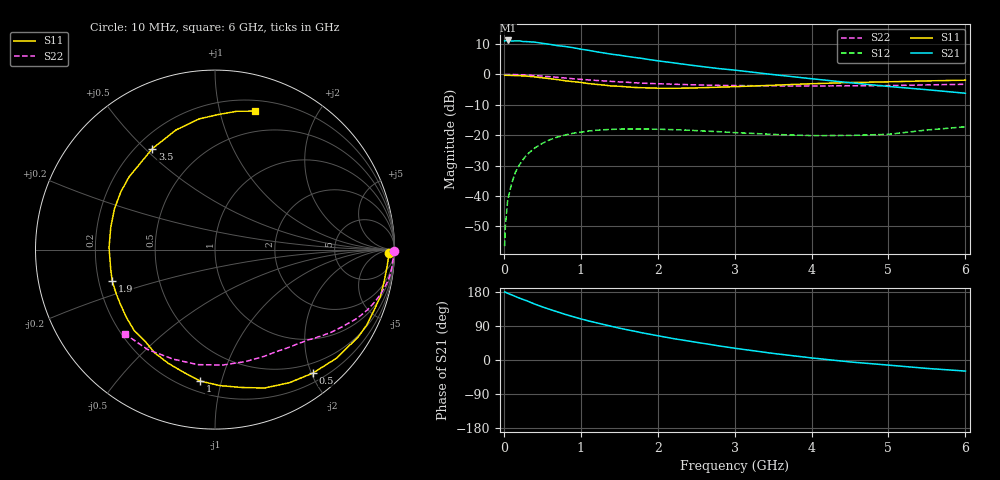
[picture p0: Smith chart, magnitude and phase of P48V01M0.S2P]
! SIEMENS Small Signal Semiconductors
! BFP182
! Si NPN RF Bipolar Junction Transistor in SOT143
! VCE = 8 V  IC = 1 mA
! Common Emitter S-Parameters:  March  1996
# GHz  S  MA  R  50
!  f  S11  S21  S12  S22
! GHz  MAG  ANG  MAG  ANG  MAG  ANG  MAG  ANG
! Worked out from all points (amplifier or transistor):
!   36 points, 10 MHz to 6 GHz, reference 50 ohm
!   highest |S21| = 11.1 dB at 50 MHz (marker M1)
!   |S21| within 3 dB of that: start of sweep to 1.037 GHz
!   unconditionally stable (mu >= 1): 2.66 GHz to end of sweep
!   at 250 MHz: K = 0.09, MSG = 19.4 dB, |S12| = -28.0 dB
!   at 1.4 GHz: K = 0.54, MSG = 12.3 dB, |S12| = -18.1 dB
!   at 6 GHz: K = 1.07, MAG = 3.9 dB, |S12| = -17.2 dB
!   S11 on the Smith chart (normalised r, x): 10 MHz: 46, -27; 500 MHz: 0.34, -2.02; 1 GHz: 0.27, -0.86; 1.9 GHz: 0.26, -0.14; 3.5 GHz: 0.26, +0.53; 6 GHz: 0.30, +1.28
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0.01  0.9683 -1.1  3.54 179.4  0.0015 89.6  0.9975 -0.4
0.02  0.9677 -2.3  3.572 179.0  0.0032 87.5  0.991 -0.7
0.05  0.9638 -5.4  3.606 175.9  0.0085 88.9  0.9965 -1.9
0.1  0.9591 -10.5  3.536 171.9  0.0159 82.1  0.9924 -4.0
0.2  0.9474 -21.4  3.553 163.5  0.0322 76.5  0.9868 -7.9
0.4  0.9079 -41.8  3.388 147.7  0.0613 64.1  0.9559 -15.1
0.5  0.8778 -51.7  3.235 140.2  0.0733 58.0  0.9348 -18.4
0.6  0.8495 -60.8  3.112 133.4  0.0844 52.9  0.9146 -21.4
0.8  0.7826 -79.0  2.869 120.3  0.101 43.0  0.8707 -26.7
1  0.7372 -96.4  2.595 108.6  0.1121 34.6  0.8281 -31.3
1.1  0.7048 -104.6  2.482 103.2  0.1172 30.9  0.8103 -33.4
1.3  0.6668 -120.2  2.246 93.6  0.1229 24.2  0.7799 -37.0
1.5  0.6376 -134.9  2.066 84.2  0.1257 18.6  0.7518 -40.3
1.9  0.5988 -162.8  1.742 67.9  0.1259 10.0  0.7089 -46.7
2.2  0.5904 178.9  1.549 56.6  0.1234 5.2  0.6885 -51.3
2.6  0.6048 157.7  1.331 43.6  0.1171 1.1  0.6662 -57.8
3  0.6273 139.7  1.174 31.1  0.1104 -1.4  0.6548 -65.2
3.5  0.6619 121.8  0.992 17.4  0.1031 -1.1  0.6464 -75.0
4  0.701 108.1  0.847 5.5  0.0985 2.6  0.6446 -86.3
4.5  0.7336 96.9  0.729 -5.1  0.0991 6.9  0.648 -98.5
5.5  0.7803 81.0  0.559 -22.2  0.1217 16.3  0.6714 -124.0
6  0.8025 74.0  0.489 -29.2  0.1376 15.2  0.687 -136.7
